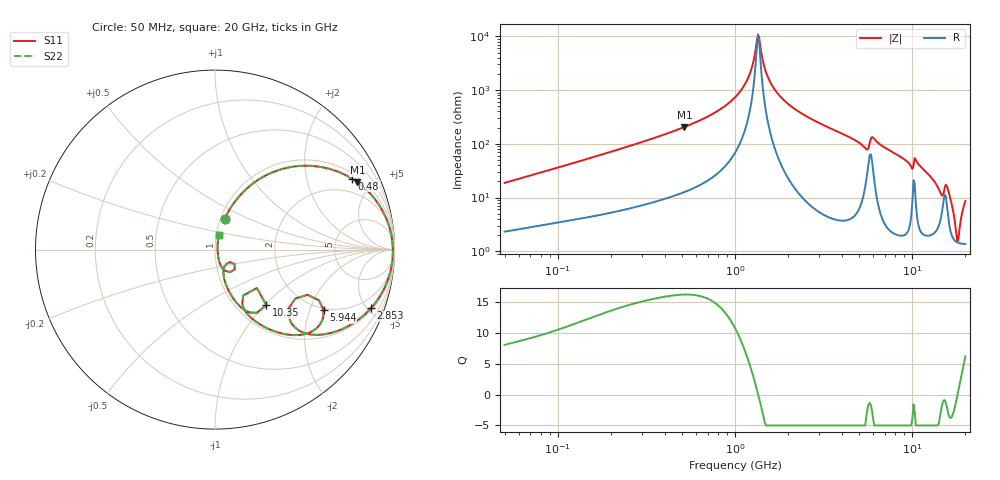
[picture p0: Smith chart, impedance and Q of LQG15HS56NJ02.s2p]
!Murata Part Number: LQG15HS56NJ02
!These Parameters are Measured in Series Mode Connection
!  o--[Z]--o
!Port1  Port2
!  o-------o
!Freq. Start=50[MHz] Stop=20[GHz], 401[Steps]
# Hz S RI R 50
!Freq.(Hz) S11(Real) S11(Imag) S21(Real) S21(Imag) S12(Real) S12(Imag) S22(Real) S22(Imag)
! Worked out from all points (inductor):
!   401 points, 50 MHz to 20 GHz, reference 50 ohm
!   read as one part in series: L = 58.4 nH near 51.52 MHz
!   highest Q = 16.2 at 517.3 MHz (marker M1), where L = 63 nH
!   self-resonance near 1.349 GHz
!   S11 on the Smith chart (normalised r, x): 50 MHz: 1.05, +0.37; 480 MHz: 1.23, +3.72; 2.853 GHz: 1.12, -5.26; 5.944 GHz: 1.94, -2.50; 10.35 GHz: 1.36, -1.02; 20 GHz: 1.03, +0.17
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5e7  0.0541 0.1724  0.9459 -0.1724  0.9459 -0.1724  0.0541 0.1724
1.364002e8  0.2119 0.3687  0.7881 -0.3687  0.7881 -0.3687  0.2119 0.3687
3.721004e8  0.6459 0.4474  0.3541 -0.4474  0.3541 -0.4474  0.6459 0.4474
4.800071e8  0.7628 0.3955  0.2372 -0.3955  0.2372 -0.3955  0.7628 0.3955
5.173368e8  0.7937 0.3749  0.2063 -0.3749  0.2063 -0.3749  0.7937 0.3749
1e9  0.97 0.1302  0.03 -0.1302  0.03 -0.1302  0.97 0.1302
1.196911e9  0.9869 0.0532  0.0131 -0.0532  0.0131 -0.0532  0.9869 0.0532
1.349283e9  0.9909 0.000847  0.00911 -0.000847  0.00911 -0.000847  0.9909 0.000847
1.498439e9  0.9895 -0.0454  0.0105 0.0454  0.0105 0.0454  0.9895 -0.0454
1.689197e9  0.9823 -0.0986  0.0177 0.0986  0.0177 0.0986  0.9823 -0.0986
2.728004e9  0.8841 -0.3085  0.1159 0.3085  0.1159 0.3085  0.8841 -0.3085
2.853386e9  0.8683 -0.327  0.1317 0.327  0.1317 0.327  0.8683 -0.327
4.608136e9  0.6032 -0.4725  0.3968 0.4725  0.3968 0.4725  0.6032 -0.4725
5.433528e9  0.424 -0.4076  0.576 0.4076  0.576 0.4076  0.424 -0.4076
5.944466e9  0.6051 -0.3356  0.3949 0.3356  0.3949 0.3356  0.6051 -0.3356
7.442007e9  0.3691 -0.4665  0.6309 0.4665  0.6309 0.4665  0.3691 -0.4665
1.034674e10  0.2864 -0.3093  0.7136 0.3093  0.7136 0.3093  0.2864 -0.3093
1.238412e10  0.083 -0.2419  0.917 0.2419  0.917 0.2419  0.083 -0.2419
1.460232e10  0.0522 -0.0966  0.9478 0.0966  0.9478 0.0966  0.0522 -0.0966
1.597544e10  0.0572 -0.118  0.9428 0.118  0.9428 0.118  0.0572 -0.118
1.800918e10  0.0144 -0.00262  0.9856 0.00262  0.9856 0.00262  0.0144 -0.00262
2e10  0.0204 0.0821  0.9796 -0.0821  0.9796 -0.0821  0.0204 0.0821
